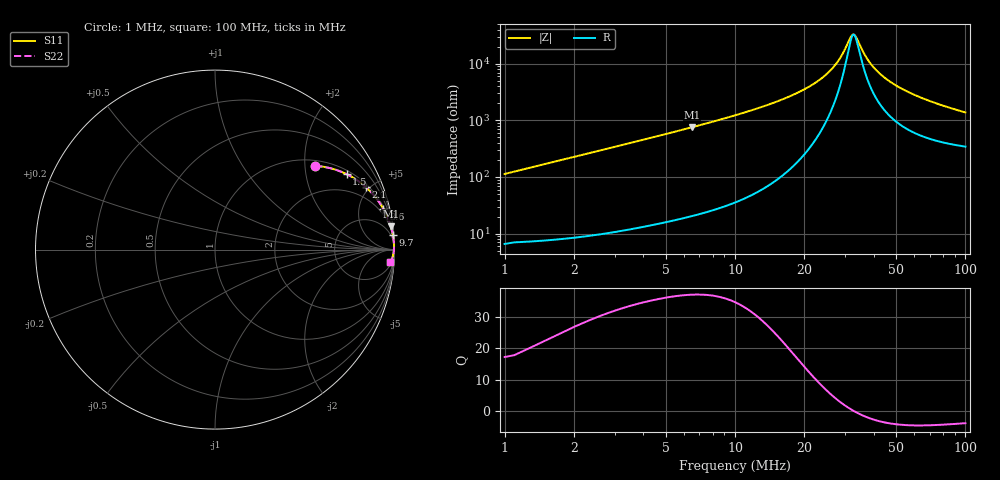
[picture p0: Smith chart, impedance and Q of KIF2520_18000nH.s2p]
!version-2
!date-12.2020
!Series
# MHz S RI R 50
!Freq ReS11 ImS11 ReS21 ImS21 ReS12 ImS12 ReS22 ImS22
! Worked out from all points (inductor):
!   991 points, 1 MHz to 100 MHz, reference 50 ohm
!   read as one part in series: L = 17.9 uH near 1.4 MHz
!   highest Q = 37 at 6.5 MHz (marker M1), where L = 18.5 uH
!   self-resonance near 32.7 MHz
!   S11 on the Smith chart (normalised r, x): 1 MHz: 1.13, +2.26; 1.5 MHz: 1.15, +3.39; 2.1 MHz: 1.17, +4.75; 3.6 MHz: 1.24, +8.18; 9.7 MHz: 2, +24; 100 MHz: 8, -27
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1  0.5587 0.4683  0.4413 -0.4683  0.4413 -0.4683  0.5587 0.4683
1.5  0.7334 0.4204  0.2666 -0.4204  0.2666 -0.4204  0.7334 0.4204
2.1  0.8408 0.3481  0.1592 -0.3481  0.1592 -0.3481  0.8408 0.3481
2.7  0.8959 0.2895  0.1041 -0.2895  0.1041 -0.2895  0.8959 0.2895
3.6  0.9376 0.2274  0.0624 -0.2274  0.0624 -0.2274  0.9376 0.2274
6.5  0.9794 0.1292  0.0206 -0.1292  0.0206 -0.1292  0.9794 0.1292
9.7  0.9906 0.0835  0.00945 -0.0835  0.00945 -0.0835  0.9906 0.0835
17.5  0.9967 0.0366  0.00327 -0.0366  0.00327 -0.0366  0.9967 0.0366
22.6  0.9974 0.0208  0.00257 -0.0208  0.00257 -0.0208  0.9974 0.0208
26.2  0.9975 0.0123  0.00255 -0.0123  0.00255 -0.0123  0.9975 0.0123
28.7  0.9973 0.00725  0.00267 -0.00725  0.00267 -0.00725  0.9973 0.00725
32.2  0.997 0.000961  0.00298 -0.000961  0.00298 -0.000961  0.997 0.000961
33  0.9969 -0.000372  0.00307 0.000372  0.00307 0.000372  0.9969 -0.000372
34  0.9968 -0.00199  0.00318 0.00199  0.00318 0.00199  0.9968 -0.00199
36.9  0.9964 -0.00644  0.00358 0.00644  0.00358 0.00644  0.9964 -0.00644
40.1  0.9959 -0.011  0.00409 0.011  0.00409 0.011  0.9959 -0.011
44.6  0.9951 -0.0168  0.00493 0.0168  0.00493 0.0168  0.9951 -0.0168
50.5  0.9938 -0.0238  0.00621 0.0238  0.00621 0.0238  0.9938 -0.0238
57.8  0.992 -0.0317  0.00803 0.0317  0.00803 0.0317  0.992 -0.0317
67  0.9893 -0.0407  0.0107 0.0407  0.0107 0.0407  0.9893 -0.0407
83.5  0.9839 -0.055  0.0161 0.055  0.0161 0.055  0.9839 -0.055
100  0.9776 -0.0674  0.0224 0.0674  0.0224 0.0674  0.9776 -0.0674
